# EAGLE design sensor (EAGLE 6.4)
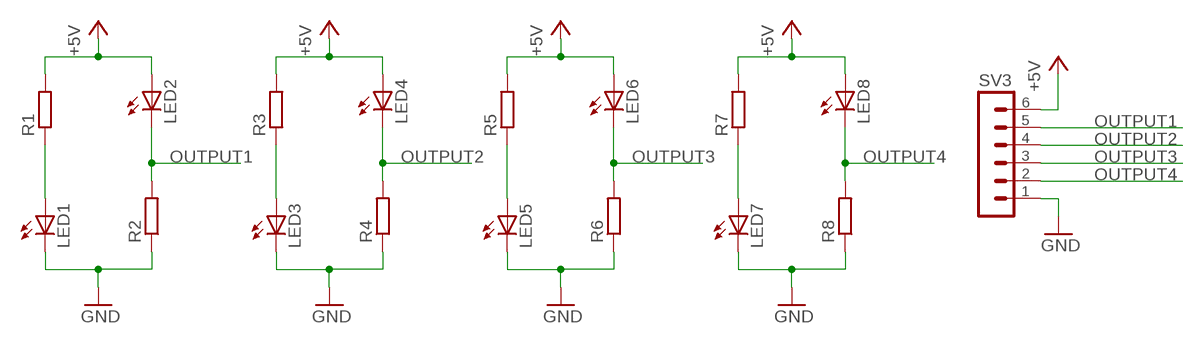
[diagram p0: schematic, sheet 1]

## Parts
LED1  LED5MM  [LED5MM]
LED2  LED5MM  [LED5MM]
LED3  LED5MM  [LED5MM]
LED4  LED5MM  [LED5MM]
LED5  LED5MM  [LED5MM]
LED6  LED5MM  [LED5MM]
LED7  LED5MM  [LED5MM]
LED8  LED5MM  [LED5MM]
R1  R-EU_0207/12  [0207/12]
R2  R-EU_0207/12  [0207/12]
R3  R-EU_0207/12  [0207/12]
R4  R-EU_0207/12  [0207/12]
R5  R-EU_0207/12  [0207/12]
R6  R-EU_0207/12  [0207/12]
R7  R-EU_0207/12  [0207/12]
R8  R-EU_0207/12  [0207/12]
SV3  MA06-1  [MA06-1]

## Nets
+5V: LED2.A LED4.A LED6.A LED8.A R1.2 R3.2 R5.2 R7.2 SV3.6
GND: LED1.K(C) LED3.K(C) LED5.K(C) LED7.K(C) R2.1 R4.1 R6.1 R8.1 SV3.1
N$1: LED3.A R3.1
N$3: LED1.A R1.1
N$5: LED5.A R5.1
N$7: LED7.A R7.1
OUTPUT1: LED2.K(C) R2.2 SV3.5
OUTPUT2: LED4.K(C) R4.2 SV3.4
OUTPUT3: LED6.K(C) R6.2 SV3.3
OUTPUT4: LED8.K(C) R8.2 SV3.2

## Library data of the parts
LED1-LED8 = led:LED: LED
R1-R8 = rcl:R-EU_: RESISTOR, European symbol
SV3 = con-lstb:MA06-1: PIN HEADER; OC_FARNELL: unknown; OC_NEWARK: unknown

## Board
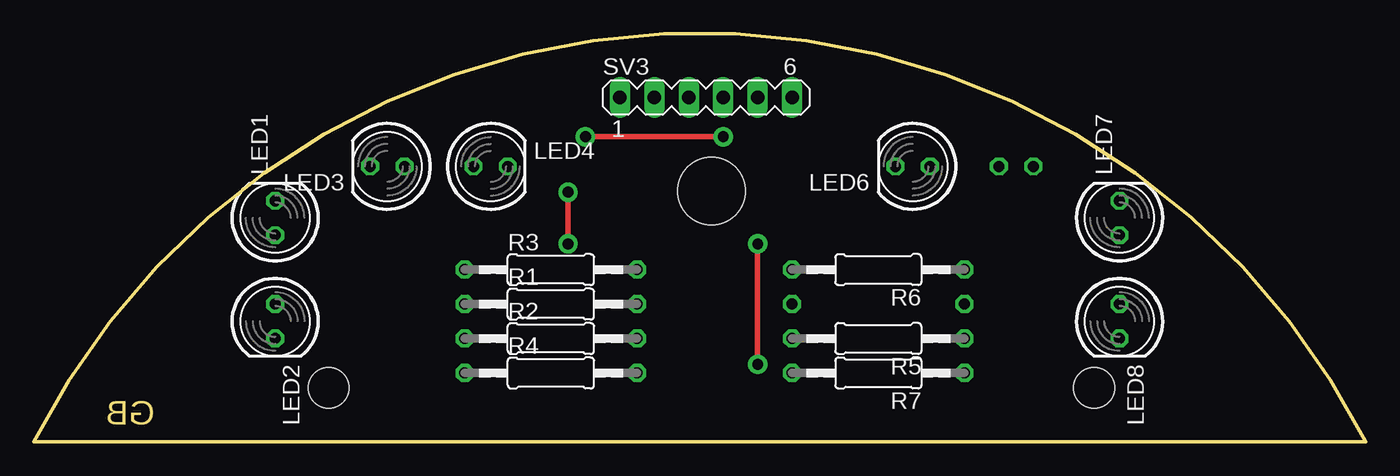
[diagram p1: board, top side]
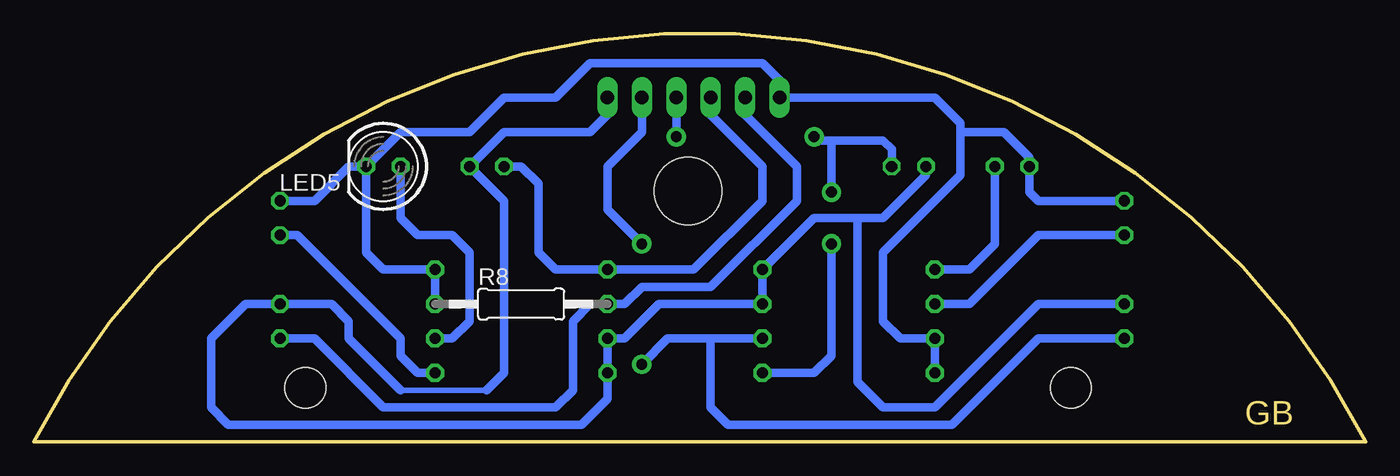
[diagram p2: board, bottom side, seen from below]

Size 98.14 x 30.09 mm. Coordinates in mm from the lower left corner, seen from the top.
Outline: 98.14,0 0,0 arc-126 98.14,0
Copper layers (1*16): Top 0.035mm / dielectric 1.5mm / Bottom 0.035mm
Design rules "default": minimum track width 10mil, minimum drill 24mil, track to track 8mil, track to pad 8mil, pad to pad 8mil, via to via 8mil, smd to smd 8mil, copper to edge 40mil, drill to drill 8mil, minimum pad ring 10mil, minimum via ring 8mil, stop-mask expansion 4mil, vias tented up to drill 0mil, thermal gap 10mil
Holes 3 mm at 78.13,3.98 21.73,3.98
Holes 5 mm at 49.93,18.49

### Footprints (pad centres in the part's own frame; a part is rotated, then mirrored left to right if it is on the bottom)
LED5MM = drill 0.813 octagon: A -1.27,0; K 1.27,0
0207/12 = drill 0.813 octagon: 1 -6.35,0; 2 6.35,0
MA06-1 = drill 1.016 long: 1 -6.35,0; 2 -3.81,0; 3 -1.27,0; 4 1.27,0; 5 3.81,0; 6 6.35,0

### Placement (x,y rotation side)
LED1  17.78,16.51 90 top
LED2  17.78,8.89 270 top
LED3  26.04,20.32 180 top
LED4  33.66,20.32 0 top
LED5  72.39,20.32 180 bottom
LED6  64.77,20.32 180 top
LED7  80.01,16.51 90 top
LED8  80.01,8.89 270 top
R1  38.1,10.16 0 top
R2  38.1,7.62 0 top
R3  38.1,12.7 0 top
R4  38.1,5.08 0 top
R5  62.23,7.62 180 top
R6  62.23,12.7 180 top
R7  62.23,5.08 180 top
R8  62.23,10.16 0 bottom
SV3  49.53,25.4 0 top

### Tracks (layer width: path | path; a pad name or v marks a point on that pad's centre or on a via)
+5V
  Bottom 0.406: 71.12,3.81 64.77,3.81
  Bottom 0.61: 71.12,3.81 74.93,7.62 74.93,8.89 76.2,10.16 LED8.A 82.55,10.16 85.09,7.62 85.09,2.54 83.82,1.27 57.78,1.27 55.88,3.17 R7.2 R5.2 54.61,7.62 52.07,10.16 R1.2 R3.2 40.64,16.51 37.47,16.51 | 64.77,3.81 63.5,5.08 63.5,17.78 LED6.A 63.5,22.86 57.15,22.86 55.88,24.13 SV3.6 | LED2.A 24.13,10.16 31.75,2.54 35.56,2.54 37.47,4.45 37.47,16.51 | LED4.A 32.38,19.68 35.56,16.51 37.47,16.51
GND
  Bottom 0.406: LED3.K 24.77,20.95
  Bottom 0.61: R8.1 R6.1 72.39,12.7 73.66,13.97 LED5.K | R4.1 R2.1 34.29,7.62 35.56,8.89 35.56,13.97 29.84,19.68 29.84,22.86 | LED5.K 71.12,22.86 66.04,22.86 63.5,25.4 59.69,25.4 57.15,27.94 44.45,27.94 43.18,26.67 SV3.1 31.75,25.4 29.84,23.5 29.84,22.86 | LED1.K 24.13,17.78 24.77,18.41 LED3.K | 24.77,20.95 26.67,22.86 29.84,22.86 | LED7.K 77.47,17.78 74.93,20.32 LED5.K
N$1
  Bottom 0.61: LED3.A 27.3,14.61 29.21,12.7 R3.1
N$3
  Bottom 0.61: LED1.A 24.13,15.24 29.21,10.16 R1.1
N$5
  Bottom 0.61: R5.1 67.31,7.62 66.04,8.89 66.04,13.97 67.31,15.24 69.85,15.24 71.12,16.51 LED5.A
N$7
  Bottom 0.61: R7.1 69.85,5.08 71.12,6.35 71.12,7.62 78.74,15.24 LED7.A
OUTPUT1  (via drill 0.8 pad 1.42)
  Top 0.406: v53.34,14.61 v53.34,5.71
  Bottom 0.61: 48.26,7.62 R2.2 | 48.26,7.62 48.26,2.54 46.99,1.27 30.48,1.27 24.13,7.62 LED2.K | 48.26,7.62 51.44,7.62 v53.34,5.71 | SV3.5 53.34,22.86 55.88,20.32 55.88,17.14 v53.34,14.61
OUTPUT2  (via drill 0.8 pad 1.42)
  Top 0.406: v40.64,22.5 v50.8,22.5 | v39.37,14.61 v39.37,18.41
  Bottom 0.61: v50.8,22.5 SV3.4 | R4.2 40.64,5.08 39.37,6.35 v39.37,14.61 | LED4.K 34.92,21.59 35.56,22.23 39.37,22.23 | 39.37,22.23 40.36,22.23 v40.64,22.5 | v39.37,18.41 39.37,22.23
OUTPUT3
  Bottom 0.61: LED6.K 62.23,20.32 60.96,19.05 60.96,13.97 59.69,12.7 R6.2 49.53,12.7 44.45,17.78 44.45,20.32 48.26,24.13 SV3.3
OUTPUT4
  Bottom 0.61: LED8.K 77.47,7.62 72.39,2.54 59.69,2.54 58.42,3.81 58.42,8.89 57.15,10.16 R8.2 54.61,10.16 53.34,11.43 48.26,11.43 41.91,17.78 41.91,20.32 45.72,24.13 SV3.2

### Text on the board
Dimension: GB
